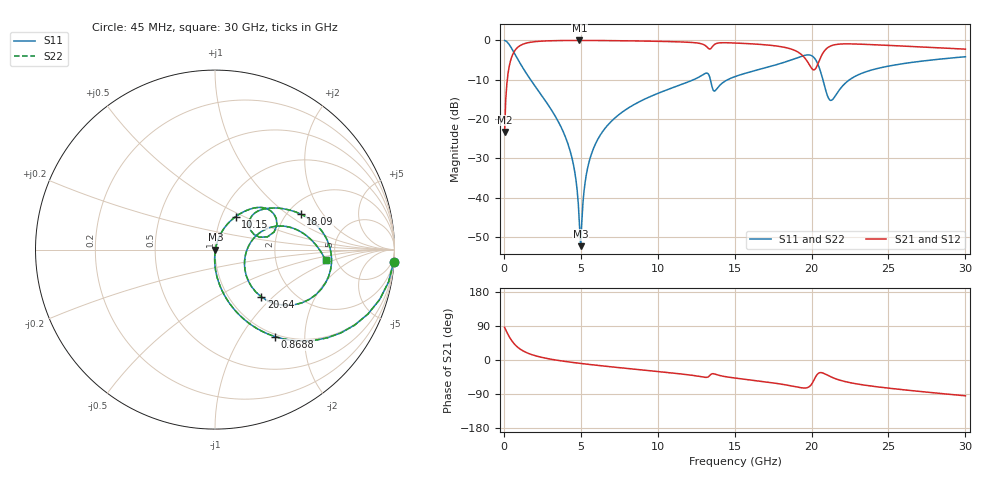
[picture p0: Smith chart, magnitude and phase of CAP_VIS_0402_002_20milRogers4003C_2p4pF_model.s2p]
! S-parameter model data by Modelithics Inc.  support@modelithics.com  813-866-6335  Tampa FL USA
! S-Parameter data specifications:
! Substrate: 20-mil Rogers 4003C, substrate thickness, H=0.508mm, Dielectric constant, Er=3.75
! PCB Mounting Pad Footprint: Pad width, PadW=0.50mm , Pad length, PadL=0.50mm , Pad gap, PadG (edge-to-edge)=0.40mm , Reference planes=1.4mm apart
! Created Wed Nov 18 12:45:33 2015
# hz S ma R 50
! 2 Port Network Data from SP1.SP block
! freq  magS11  angS11  magS21  angS21  magS12  angS12  magS22  angS22
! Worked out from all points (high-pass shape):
!   401 points, 45 MHz to 30 GHz, reference 50 ohm
!   highest |S21| = -0.02 dB at 4.913 GHz (marker M1); lowest = -23.3 dB at 45 MHz (marker M2)
!   |S21| within 3 dB of the highest: 644 MHz to 19.14 GHz (18.49 GHz wide, 187 % of centre); 20.77 GHz to end of sweep
!   lowest |S11| = -52.4 dB at 4.988 GHz (marker M3), VSWR 1.00, Z = 50.2 - j0.0157 ohm
!   |S11| at or under -10 dB: 1.732 GHz to 12.33 GHz (10.6 GHz wide, 151 % of centre); 13.42 GHz to 14.55 GHz (1.128 GHz wide, 8.06 % of centre); 20.74 GHz to 22.48 GHz (1.741 GHz wide, 8.06 % of centre)
!   |S22| runs from -52.4 to 0.0 dB; largest |S21 - S12| = 0
!   S11 on the Smith chart (normalised r, x): 45 MHz: 1, -29; 868.8 MHz: 0.96, -1.44; 10.15 GHz: 1.17, +0.45; 18.09 GHz: 2.34, +1.27; 20.64 GHz: 1.39, -0.85; 30 GHz: 4.09, -0.79
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4.5e7  0.9977 -4.0  0.06846 86.0  0.06846 86.0  0.9977 -4.0
3.4455e8  0.8842 -28.5  0.4667 61.5  0.4667 61.5  0.8842 -28.5
8.687625e8  0.5905 -55.3  0.8062 34.6  0.8062 34.6  0.5905 -55.3
1.8423e9  0.2941 -76.0  0.9543 13.7  0.9543 13.7  0.2941 -76.0
4.014038e9  0.0579 -91.9  0.9961 -4.0  0.9961 -4.0  0.0579 -91.9
4.53825e9  0.02509 -91.6  0.9973 -6.8  0.9973 -6.8  0.02509 -91.6
4.912688e9  0.004499 -66.8  0.9975 -8.7  0.9975 -8.7  0.004499 -66.8
4.987575e9  0.002406 -3.7  0.9975 -9.1  0.9975 -9.1  0.002406 -3.7
5.062462e9  0.004858 50.7  0.9974 -9.5  0.9974 -9.5  0.004858 50.7
5.511788e9  0.02723 73.1  0.9969 -11.6  0.9969 -11.6  0.02723 73.1
6.260662e9  0.06219 72.5  0.9952 -15.0  0.9952 -15.0  0.06219 72.5
1.007992e10  0.2145 58.2  0.9723 -30.7  0.9723 -30.7  0.2145 58.2
1.015481e10  0.2174 57.9  0.9716 -31.0  0.9716 -31.0  0.2174 57.9
1.307542e10  0.3786 34.6  0.8634 -45.7  0.8634 -45.7  0.3786 34.6
1.352475e10  0.2591 15.3  0.8181 -36.4  0.8181 -36.4  0.2591 15.3
1.50225e10  0.346 40.3  0.9254 -47.6  0.9254 -47.6  0.346 40.3
1.809289e10  0.5163 22.6  0.8264 -64.1  0.8264 -64.1  0.5163 22.6
2.003996e10  0.6329 -20.1  0.4324 -61.4  0.4324 -61.4  0.6329 -20.1
2.063906e10  0.3693 -45.6  0.6354 -33.3  0.6354 -33.3  0.3693 -45.6
2.131305e10  0.1735 -5.9  0.8594 -45.5  0.8594 -45.5  0.1735 -5.9
2.505742e10  0.4728 13.3  0.8624 -74.5  0.8624 -74.5  0.4728 13.3
3e10  0.619 -5.5  0.7728 -94.5  0.7728 -94.5  0.619 -5.5
